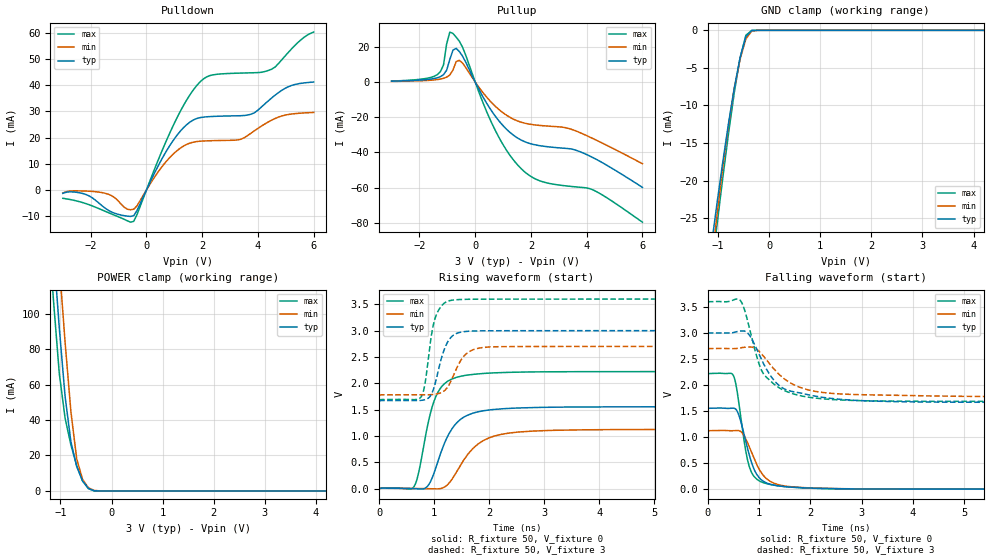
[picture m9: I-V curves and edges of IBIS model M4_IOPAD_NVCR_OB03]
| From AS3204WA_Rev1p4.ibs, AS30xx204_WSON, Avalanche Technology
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[Model] M4_IOPAD_NVCR_OB03
Model_type I/O
Enable   Active-High
Vinl  =  0.9
Vinh  =  2.1
Vmeas =  1.5
Cref  =  30e-12
| Capacitance  typ   min   max
C_comp   3.872127e-12   3.590660e-12   4.176448e-12
| Variables   typ   min   max
[GND Clamp Reference]   0   0   0
[POWER Clamp Reference]   3   2.7   3.6
[Pulldown Reference]   0   0   0
[Pullup Reference]   3   2.7   3.6
[Temperature Range]   25   105   -40
[Voltage Range]   3   2.7   3.6
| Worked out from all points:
|   slope of the pulldown table from 0 to 0.45 V, typ, clamps not added: 46 ohm
|   slope of the pullup table from 0 to 0.45 V, typ, clamps not added: 34.5 ohm
|   GND clamp passes 1 mA (typ) near -0.46 V on its own axis
|   POWER clamp passes 1 mA (typ) near -0.42 V on its own axis
|   falling waveform, R_fixture 50, V_fixture 0: 20-80 % time 279ps typ, 349ps min, 219ps max; typ from 1.55 V to 0 V
|   falling waveform, R_fixture 50, V_fixture 3: 20-80 % time 543ps typ, 663ps min, 453ps max; typ from 3 V to 1.67 V
|   rising waveform, R_fixture 50, V_fixture 0: 20-80 % time 402ps typ, 521ps min, 297ps max; typ from 0 V to 1.55 V
|   rising waveform, R_fixture 50, V_fixture 3: 20-80 % time 219ps typ, 276ps min, 166ps max; typ from 1.67 V to 3 V
[GND Clamp]
| Voltage   I(typ)   I(min)   I(max)
-3V       -145.9mA   -151.9mA   -144.2mA
-1.138V   -29.07mA   -31.55mA   -32.68mA
-1.024V   -23.24mA   -24.83mA   -26.15mA
-910.3mV  -17.69mA   -18.46mA   -19.83mA
-796.6mV  -12.47mA   -12.67mA   -13.82mA
-682.8mV  -7.718mA   -7.754mA   -8.316mA
-569mV    -3.663mA   -3.867mA   -3.675mA
-455.2mV  -839.2uA   -1.152mA   -666.1uA
-341.4mV  -35.63uA   -111.1uA   -11.17uA
-113.8mV  -8.642nA   -188.3nA   -1.888nA
6V        0A         0A         0A
[POWER Clamp]
| Voltage   I(typ)   I(min)   I(max)
-3V       949.8mA    984.2mA    923.5mA
-1.252V   183.6mA    221.4mA    154mA
-1.138V   136.7mA    174.2mA    107.6mA
-1.024V   92.09mA    128.1mA    66.35mA
-910.3mV  53.33mA    83.97mA    41.06mA
-796.6mV  27.72mA    44.75mA    25.94mA
-682.8mV  13.75mA    18.06mA    14.29mA
-569mV    5.664mA    6.605mA    5.738mA
-455.2mV  1.446mA    1.789mA    1.305mA
-341.4mV  77.09uA    287.6uA    62.73uA
-227.6mV  1.148uA    12.92uA    332nA
6V        0A         0A         0A
[Pulldown]
| Voltage   I(typ)   I(min)   I(max)
-3V       -1.302mA   -1.149mA   -3.185mA
-2.162V   -1.762mA   -423uA     -5.24mA
-1.479V   -6.973mA   -1.259mA   -8.151mA
-455.2mV  -9.808mA   -7.331mA   -11.97mA
931mV     18.47mA    13.42mA    23.93mA
1.862V    27.49mA    18.57mA    40.59mA
2.379V    28.09mA    18.84mA    43.96mA
3.372V    28.37mA    19.32mA    44.65mA
3.745V    28.91mA    21.64mA    44.76mA
4.49V     35.12mA    26.66mA    46.12mA
5.11V     39.54mA    28.87mA    52.79mA
6V        41.23mA    29.62mA    60.32mA
[Pullup]
| Voltage   I(typ)   I(min)   I(max)
-3V       480.5uA    358.7uA    563.8uA
-1.366V   2.392mA    1.388mA    4.137mA
-1.138V   4.176mA    2.092mA    9.68mA
-910.3mV  12.91mA    4.004mA    28.39mA
-796.6mV  18.14mA    6.858mA    27.6mA
-569mV    17.36mA    12.34mA    23.19mA
620.7mV   -17.18mA   -12.21mA   -24.25mA
1.655V    -33.03mA   -22.87mA   -49.34mA
2.379V    -36.33mA   -24.76mA   -56.49mA
3.745V    -39.52mA   -28.67mA   -59.79mA
4.366V    -44.12mA   -33.21mA   -62.42mA
6V        -59.9mA    -46.44mA   -79.67mA
[Ramp]
dV/dt_r   0.931955/0.401817n  0.673943/0.520651n  1.33324/0.296908n
dV/dt_f   0.799473/0.543284n  0.553656/0.663318n  1.14844/0.452872n
R_load = 50
[Falling Waveform]
R_fixture = 50
V_fixture = 0
V_fixture_min = 0
V_fixture_max = 0
| Time   V(typ)   V(min)   V(max)
0s        1.553V     1.123V     2.222V
495.5ps   1.556V     1.123V     2.189V
543ps     1.539V     1.126V     2.038V
615.3ps   1.394V     1.121V     1.583V
731.8ps   952.6mV    982.6mV    780.2mV
838.4ps   555.3mV    741.3mV    354.5mV
949.5ps   291.5mV    484.3mV    196.4mV
1.101ns   140.7mV    243.8mV    118.6mV
1.489ns   50.53mV    63.13mV    50.77mV
21.88ns   478.9nV    595.3nV    10.18uV
[Falling Waveform]
R_fixture = 50
V_fixture = 3
V_fixture_min = 2.7
V_fixture_max = 3.6
| Time   V(typ)   V(min)   V(max)
0s        3V         2.7V       3.6V
625.8ps   3.037V     2.712V     3.633V
699.1ps   3.039V     2.724V     3.498V
813.3ps   2.956V     2.731V     3.087V
978.9ps   2.635V     2.668V     2.466V
1.092ns   2.4V       2.547V     2.205V
1.459ns   1.943V     2.145V     1.911V
2.195ns   1.77V      1.864V     1.738V
4.389ns   1.672V     1.79V      1.687V
21.88ns   1.668V     1.777V     1.686V
[Rising Waveform]
R_fixture = 50
V_fixture = 0
V_fixture_min = 0
V_fixture_max = 0
| Time   V(typ)   V(min)   V(max)
0s        382nV      443.2nV    10.07uV
614.8ps   -1.423mV   3.059mV    9.209mV
711ps     -7.837mV   1.293mV    263.7mV
872.8ps   33.79mV    -3.33mV    1.152V
1.07ns    516.4mV    -7.116mV   1.829V
1.361ns   1.187V     233.3mV    2.096V
1.693ns   1.428V     746.7mV    2.168V
2.226ns   1.515V     1.03V      2.203V
3.482ns   1.548V     1.112V     2.22V
21.88ns   1.553V     1.123V     2.222V
[Rising Waveform]
R_fixture = 50
V_fixture = 3
V_fixture_min = 2.7
V_fixture_max = 3.6
| Time   V(typ)   V(min)   V(max)
0s        1.668V     1.777V     1.686V
767.9ps   1.675V     1.779V     1.744V
837.4ps   1.689V     1.779V     2.007V
933.6ps   1.761V     1.783V     2.787V
1.032ns   2.045V     1.794V     3.278V
1.196ns   2.673V     1.865V     3.53V
1.389ns   2.938V     2.237V     3.587V
1.655ns   2.991V     2.612V     3.596V
2.199ns   2.998V     2.696V     3.599V
21.88ns   3V         2.7V       3.6V
